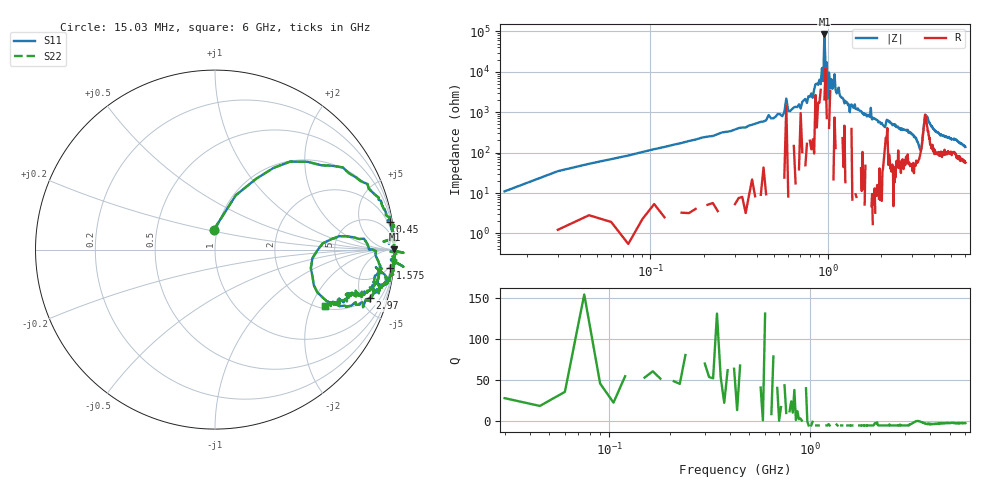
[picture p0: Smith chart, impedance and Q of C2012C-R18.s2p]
!	Network	Analyzer	HP8753E.07.74:	Oct	30	2002	Serial	No.	JP38451487
!	Hewlett-Packard
!	7	Sep	2009	12:16:19
!	Frequency	S11	S21	S12	S22
#	HZ	S	RI	R	50
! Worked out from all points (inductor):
!   400 points, 15.03 MHz to 6 GHz, reference 50 ohm
!   read as one part in series: L = 182 nH near 45.03 MHz
!   highest |Z| = 84 kohm at 960 MHz (marker M1)
!   self-resonance near 960 MHz
!   S11 on the Smith chart (normalised r, x): 15.03 MHz: 0.96, +0.22; 450 MHz: 1, +13; 1.575 GHz: 3, -18; 2.97 GHz: 1.99, -5.92; 6 GHz: 2.12, -2.52
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1.502992e7  -0.00665 0.111  1.01 -0.111  1.01 -0.111  -0.00665 0.111
9.002955e7  0.516 0.489  0.484 -0.489  0.484 -0.489  0.516 0.489
4.500278e8  0.973 0.154  0.0267 -0.154  0.0267 -0.154  0.973 0.154
5.850271e8  0.969 0.0319  0.0309 -0.0319  0.0309 -0.0319  0.969 0.0319
8.250259e8  0.994 0.0434  0.00601 -0.0434  0.00601 -0.0434  0.994 0.0434
9.300254e8  1 0.00812  -0.00012 -0.00812  -0.00012 -0.00812  1 0.00812
9.450253e8  1.01 0.0108  -0.0133 -0.0108  -0.0133 -0.0108  1.01 0.0108
9.600252e8  1 0.00119  3.1e-05 -0.00119  3.1e-05 -0.00119  1 0.00119
9.750251e8  0.993 -0.00208  0.00748 0.00208  0.00748 0.00208  0.993 -0.00208
9.90025e8  1 -0.0058  0.000275 0.0058  0.000275 0.0058  1 -0.0058
1.005025e9  1.05 -0.0174  -0.045 0.0174  -0.045 0.0174  1.05 -0.0174
1.020025e9  0.999 -0.0104  0.00055 0.0104  0.00055 0.0104  0.999 -0.0104
1.335023e9  1.05 -0.095  -0.0462 0.095  -0.0462 0.095  1.05 -0.095
1.575022e9  0.977 -0.103  0.0227 0.103  0.0227 0.103  0.977 -0.103
2.01002e9  0.962 -0.178  0.0378 0.178  0.0378 0.178  0.962 -0.178
2.970015e9  0.864 -0.269  0.136 0.269  0.136 0.269  0.864 -0.269
3.015015e9  0.864 -0.287  0.136 0.287  0.136 0.287  0.864 -0.287
3.360013e9  0.534 -0.103  0.466 0.103  0.466 0.103  0.534 -0.103
3.555012e9  0.897 -0.00885  0.103 0.00885  0.103 0.00885  0.897 -0.00885
4.00501e9  0.879 -0.22  0.121 0.22  0.121 0.22  0.879 -0.22
5.010005e9  0.745 -0.254  0.255 0.254  0.255 0.254  0.745 -0.254
6e9  0.612 -0.313  0.388 0.313  0.388 0.313  0.612 -0.313
